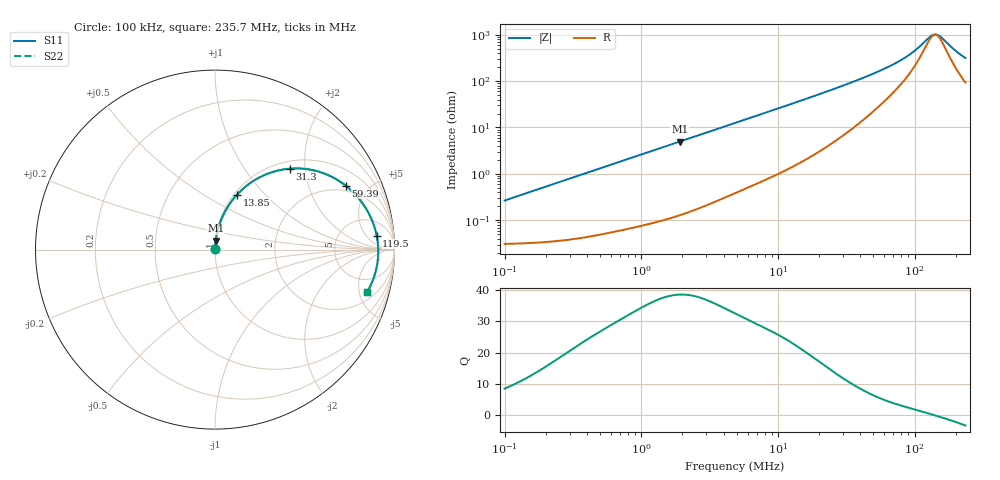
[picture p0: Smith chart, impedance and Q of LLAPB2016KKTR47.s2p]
! LLAPB2016KKTR47  S-PARAMETER MODEL  ( General Type )
! Model Generated by TAIYO YUDEN Corporation (http://www.ty-top.com)
! Version 2.0
! TAIYO YUDEN Control No. 20210629
! Copyright(c) 2015 TAIYO YUDEN CO.,LTD. All Rights Reserved.
! Product Description (link to TY-COMPAS)
! https://ds.yuden.co.jp/TYCOMPAS/or/detail?pn=LLAPB2016KKTR47M&u=M
! Products Name : Inductors
! Characteristics :
!  Inductance : 0.47 uH , SRF(min) : -Hz , DC Resistance(max) : 0.036 Ohm
!  Rated Current : Saturation :4300 mA , Temp Rise : 3300 mA (40 degC)
!  Case Size : 2.0 x 1.6 / 0.079 x 0.063 [mm/inch] , Thickness : 1 / 0.039 [mm/inch]
!  (Conditions: Temperature = 25 degC , DC Bias Current/Voltage = 0A / 0V)
! External Node Assignments :
!  1  o---GGG---o  2
! GND o---------o GND
! Frequency Range : 0.1MHz  -  235.669543MHz  [ 402 STEP ]
# MHz S RI R 50
! Freq[MHz].  S11 Real  S11 Imag  S21 Real  S21 Imag  S12 Real  S12 Imag  S22 Real  S22 Imag
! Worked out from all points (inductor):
!   401 points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, 100 kHz to 235.7 MHz, reference 50 ohm
!   read as one part in series: L = 423 nH near 104 kHz
!   highest Q = 38.6 at 1.912 MHz (marker M1), where L = 414 nH
!   self-resonance near 141.4 MHz
!   S11 on the Smith chart (normalised r, x): 100 kHz: 1.00, +0.01; 13.85 MHz: 1.03, +0.71; 31.3 MHz: 1.15, +1.66; 59.39 MHz: 1.71, +3.55; 119.5 MHz: 11, +10; 235.7 MHz: 2.86, -5.98
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0.1  0.000318 0.00266  0.9997 -0.00266  0.9997 -0.00266  0.000318 0.00266
0.367165  0.000514 0.0097  0.9995 -0.0097  0.9995 -0.0097  0.000514 0.0097
1.348099  0.00218 0.035  0.9978 -0.035  0.9978 -0.035  0.00218 0.035
1.911945  0.00374 0.0494  0.9963 -0.0494  0.9963 -0.0494  0.00374 0.0494
4.854581  0.019 0.1221  0.981 -0.1221  0.981 -0.1221  0.019 0.1221
8.861459  0.0561 0.2123  0.9439 -0.2123  0.9439 -0.2123  0.0561 0.2123
13.84882  0.1229 0.3064  0.8771 -0.3064  0.8771 -0.3064  0.1229 0.3064
17.8243  0.1872 0.3643  0.8128 -0.3643  0.8128 -0.3643  0.1872 0.3643
23.3907  0.2842 0.4191  0.7158 -0.4191  0.7158 -0.4191  0.2842 0.4191
31.29713  0.4183 0.4511  0.5817 -0.4511  0.5817 -0.4511  0.4183 0.4511
42.69694  0.5773 0.4345  0.4227 -0.4345  0.4227 -0.4345  0.5773 0.4345
59.39086  0.7282 0.3562  0.2718 -0.3562  0.2718 -0.3562  0.7282 0.3562
65.44454  0.7648 0.3243  0.2352 -0.3243  0.2352 -0.3243  0.7648 0.3243
91.03246  0.8588 0.1975  0.1412 -0.1975  0.1412 -0.1975  0.8588 0.1975
104.2825  0.884 0.1392  0.116 -0.1392  0.116 -0.1392  0.884 0.1392
119.4612  0.9009 0.0782  0.0991 -0.0782  0.0991 -0.0782  0.9009 0.0782
134.2182  0.9084 0.0243  0.0916 -0.0243  0.0916 -0.0243  0.9084 0.0243
142.2669  0.9097 -0.00294  0.0903 0.00294  0.0903 0.00294  0.9097 -0.00294
147.899  0.9096 -0.0212  0.0904 0.0212  0.0904 0.0212  0.9096 -0.0212
159.841  0.9071 -0.0578  0.0929 0.0578  0.0929 0.0578  0.9071 -0.0578
201.7704  0.881 -0.1667  0.119 0.1667  0.119 0.1667  0.881 -0.1667
235.6695  0.8475 -0.2361  0.1525 0.2361  0.1525 0.2361  0.8475 -0.2361
